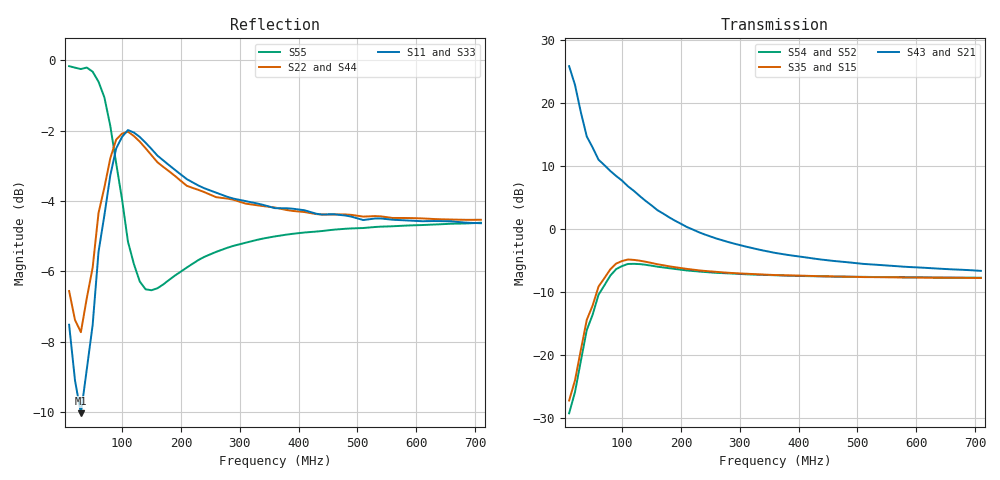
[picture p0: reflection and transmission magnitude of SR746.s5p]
!  POLYFET RF DEVICES
!  SR746
!  (Each side)
!  S PARAMETERS
!  VDS=50V, IDQ=400mA
!AWR Design Environment (2053) Wed Feb 04 15:54:20 2004
!freq-unit  param-type  data-format  keyword  impedance-ohms
# MHz  S  MA  R  50
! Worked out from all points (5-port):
!   71 points, 10 MHz to 710 MHz, reference 50 ohm
!   strongest paths, dB at 10 MHz, 180 MHz, 360 MHz, 540 MHz, 710 MHz:
!     S43: 25.8, 1.8, -3.8, -5.8, -6.7
!     S21: 25.8, 1.8, -3.8, -5.8, -6.7
!     S35: -27.2, -5.9, -7.3, -7.7, -7.8
!     S15: -27.2, -5.9, -7.3, -7.7, -7.8
!     S54: -29.3, -6.3, -7.4, -7.7, -7.8
!     S52: -29.3, -6.3, -7.4, -7.7, -7.8
!   lowest |S11| = -10.0 dB at 30 MHz (marker M1), VSWR 1.92, Z = 51.2 - j33.5 ohm
!   |S11| at or under -10 dB: 29.54 MHz to 30.34 MHz (801.8 kHz wide, 2.68 % of centre)
